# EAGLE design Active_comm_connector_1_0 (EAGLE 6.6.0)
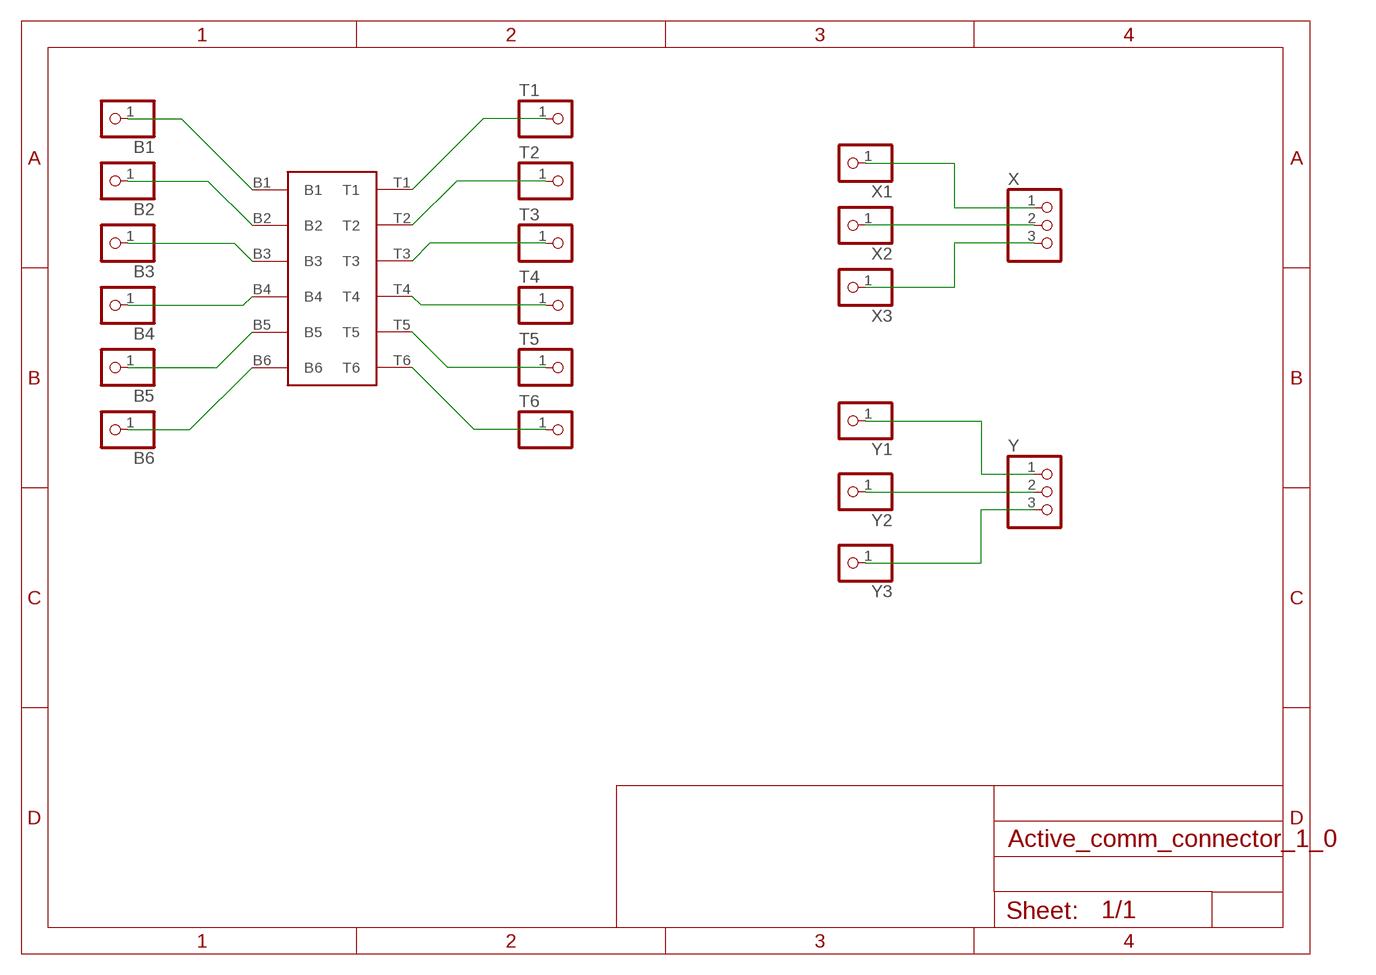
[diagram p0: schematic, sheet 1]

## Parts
B1  PINHD-1X1  [1X01]
B2  PINHD-1X1  [1X01]
B3  PINHD-1X1  [1X01]
B4  PINHD-1X1  [1X01]
B5  PINHD-1X1  [1X01]
B6  PINHD-1X1  [1X01]
PZN-12-VV  PZN-12-VV  [OMNETICS_PZN-12-VV]
T1  PINHD-1X1  [1X01]
T2  PINHD-1X1  [1X01]
T3  PINHD-1X1  [1X01]
T4  PINHD-1X1  [1X01]
T5  PINHD-1X1  [1X01]
T6  PINHD-1X1  [1X01]
X  PINHD-1X3  [1X03]
X1  PINHD-1X1  [1X01]
X2  PINHD-1X1  [1X01]
X3  PINHD-1X1  [1X01]
Y  PINHD-1X3  [1X03]
Y1  PINHD-1X1  [1X01]
Y2  PINHD-1X1  [1X01]
Y3  PINHD-1X1  [1X01]

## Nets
B4: B4.1 PZN-12-VV.B4
N$1: B1.1 PZN-12-VV.B1
N$2: B2.1 PZN-12-VV.B2
N$3: B3.1 PZN-12-VV.B3
N$4: Y1.1 Y.1
N$5: B5.1 PZN-12-VV.B5
N$6: B6.1 PZN-12-VV.B6
N$7: PZN-12-VV.T1 T1.1
N$8: PZN-12-VV.T2 T2.1
N$9: PZN-12-VV.T3 T3.1
N$10: PZN-12-VV.T4 T4.1
N$11: PZN-12-VV.T5 T5.1
N$12: PZN-12-VV.T6 T6.1
N$13: Y2.1 Y.2
N$14: Y3.1 Y.3
N$16: X2.1 X.2
N$17: X3.1 X.3
XX1: X1.1 X.1

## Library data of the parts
B1-B6 T1-T6 X1-X3 Y1-Y3 = adafruit:PINHD-1X1: Pin header 1x1 for 0.1" spacing
PZN-12-VV = omnetics_con:PZN-12-VV
X Y = adafruit:PINHD-1X3: PIN HEADER

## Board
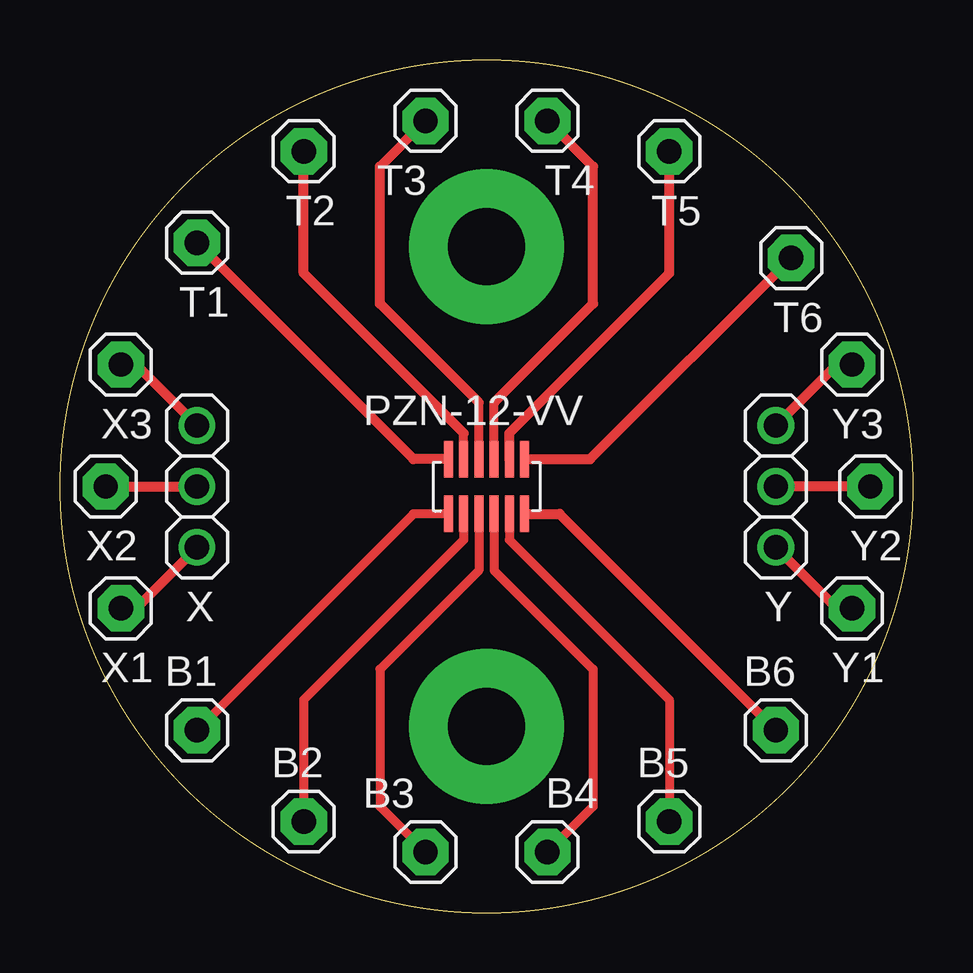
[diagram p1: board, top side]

Size 35.56 x 35.56 mm. Coordinates in mm from the lower left corner, seen from the top.
Outline: circle at 17.78,17.78 radius 17.78
Copper layers (1*16): Top 0.035mm / dielectric 1.5mm / Bottom 0.035mm
Design rules "default": minimum track width 10mil, minimum drill 24mil, track to track 8mil, track to pad 8mil, pad to pad 8mil, via to via 8mil, smd to smd 8mil, copper to edge 40mil, drill to drill 8mil, minimum pad ring 10mil, minimum via ring 8mil, stop-mask expansion 4mil, vias tented up to drill 0mil, thermal gap 10mil

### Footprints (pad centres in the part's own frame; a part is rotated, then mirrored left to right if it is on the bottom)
1X01 = drill 1.016 pad 1.93 octagon: 1 0,0
OMNETICS_PZN-12-VV = smd 0.381 x 1.524: B1 1.587,1.143; B2 0.953,1.143; B3 0.318,1.143; B4 -0.318,1.143; B5 -0.953,1.143; B6 -1.587,1.143; T1 1.587,-1.143; T2 0.953,-1.143; T3 0.318,-1.143; T4 -0.318,-1.143; T5 -0.953,-1.143; T6 -1.587,-1.143
1X03 = drill 1.016: 1 -2.54,0; 2 0,0; 3 2.54,0

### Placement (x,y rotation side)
B1  5.71,7.62 0 top
B2  10.16,3.81 0 top
B3  15.24,2.54 0 top
B4  20.32,2.54 0 top
B5  25.4,3.81 0 top
B6  29.84,7.62 0 top
PZN-12-VV  17.78,17.78 180 top
T1  5.71,27.94 180 top
T2  10.16,31.75 180 top
T3  15.24,33.02 180 top
T4  20.32,33.02 180 top
T5  25.4,31.75 180 top
T6  30.48,27.3 180 top
X  5.71,17.78 90 top
X1  2.54,12.7 180 top
X2  1.91,17.78 180 top
X3  2.54,22.86 180 top
Y  29.84,17.78 90 top
Y1  33.02,12.7 180 top
Y2  33.78,17.78 180 top
Y3  33.02,22.86 180 top

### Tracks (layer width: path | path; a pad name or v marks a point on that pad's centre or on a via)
B4
  Top 0.381: PZN-12-VV.B4 18.1,14.29 22.23,10.16 22.23,4.45 B4.1
N$1
  Top 0.381: PZN-12-VV.B1 14.73,16.64 B1.1
N$2
  Top 0.381: PZN-12-VV.B2 16.83,15.56 10.16,8.89 B2.1
N$3
  Top 0.381: PZN-12-VV.B3 17.46,14.29 13.34,10.16 13.34,4.45 B3.1
N$4
  Top 0.406: Y1.1 32.38,12.7 Y.1
N$5
  Top 0.381: PZN-12-VV.B5 18.73,15.56 25.4,8.89 B5.1
N$6
  Top 0.406: PZN-12-VV.B6 20.83,16.64 B6.1
N$7
  Top 0.406: PZN-12-VV.T1 14.73,18.92 T1.1
N$8
  Top 0.381: PZN-12-VV.T2 16.83,20
  Top 0.406: 16.83,20 10.16,26.67 T2.1
N$9
  Top 0.381: PZN-12-VV.T3 17.46,21.27
  Top 0.406: 17.46,21.27 13.34,25.4 13.34,31.11 T3.1
N$10
  Top 0.381: PZN-12-VV.T4 18.1,21.27
  Top 0.406: 18.1,21.27 22.23,25.4 22.23,31.11 T4.1
N$11
  Top 0.406: PZN-12-VV.T5 18.73,20 25.4,26.67 T5.1
N$12
  Top 0.406: PZN-12-VV.T6 22.1,18.92 T6.1
N$13
  Top 0.406: Y2.1 Y.2
N$14
  Top 0.406: Y3.1 32.38,22.86 Y.3
N$16
  Top 0.406: X2.1 X.2
N$17
  Top 0.406: X3.1 3.17,22.86 X.3
N$18  (via drill 3.2 pad 6.45)
  other vias: 17.78,7.78
N$19  (via drill 3.2 pad 6.45)
  other vias: 17.78,27.78
XX1
  Top 0.406: X1.1 3.17,12.7 X.1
